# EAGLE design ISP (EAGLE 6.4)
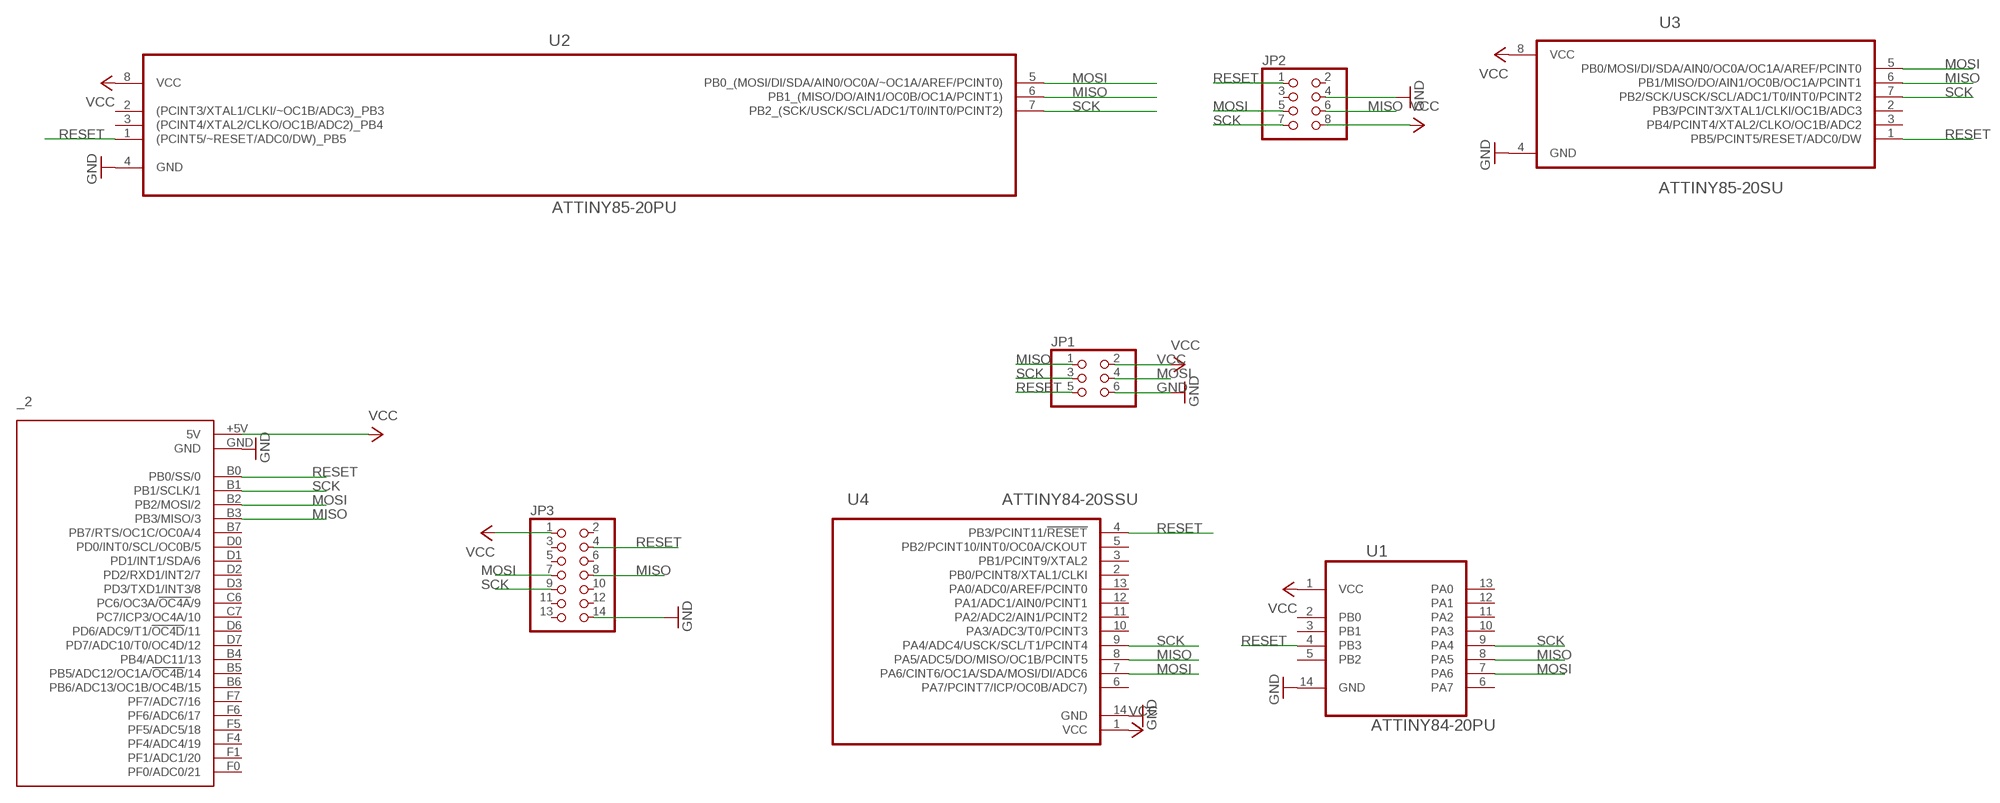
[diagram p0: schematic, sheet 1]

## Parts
_2  TEENSY-OUTER  [TEENSY-OUTER]
JP1  PINHD-2X3  [2X03]
JP2  PINHD-2X4  [2X04]
JP3  PINHD-2X7  [2X07]
U1  ATTINY84-20PU  [DIP254P762X533-14]
U2  ATTINY85-20PU  [DIP254P762X533-8]
U3  ATTINY85-20SU  [SOIC127P798X216-8N]
U4  ATTINY84-20SSU  [SOIC127P600X175-14N]

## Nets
GND: _2.GND JP1.6 JP2.4 JP3.14 U1.14(GND) U2.4(GND) U3.4(GND) U4.14(GND)
MISO: _2.B3(PB3/MISO/3) JP1.1 JP2.6 JP3.8 U1.8(PA5) U2.6(PB1_(MISO/DO/AIN1/OC0B/OC1A/PCINT1)) U3.6(PB1/MISO/DO/AIN1/OC0B/OC1A/PCINT1) U4.8(PA5/ADC5/DO/MISO/OC1B/PCINT5)
MOSI: _2.B2(PB2/MOSI/2) JP1.4 JP2.5 JP3.7 U1.7(PA6) U2.5(PB0_(MOSI/DI/SDA/AIN0/OC0A/~OC1A/AREF/PCINT0)) U3.5(PB0/MOSI/DI/SDA/AIN0/OC0A/OC1A/AREF/PCINT0) U4.7(PA6/CINT6/OC1A/SDA/MOSI/DI/ADC6)
RESET: _2.B0(PB0/SS/0) JP1.5 JP2.1 JP3.4 U1.4(PB3) U2.1((PCINT5/~RESET/ADC0/DW)_PB5) U3.1(PB5/PCINT5/RESET/ADC0/DW) U4.4(PB3/PCINT11/!RESET)
SCK: _2.B1(PB1/SCLK/1) JP1.3 JP2.7 JP3.9 U1.9(PA4) U2.7(PB2_(SCK/USCK/SCL/ADC1/T0/INT0/PCINT2)) U3.7(PB2/SCK/USCK/SCL/ADC1/T0/INT0/PCINT2) U4.9(PA4/ADC4/USCK/SCL/T1/PCINT4)
VCC: _2.+5V(5V) JP1.2 JP2.8 JP3.1 U1.1(VCC) U2.8(VCC) U3.8(VCC) U4.1(VCC)
Unconnected: _2.B4(PB4/ADC11/13) _2.B5(PB5/ADC12/OC1A/!OC4B!/14) _2.B6(PB6/ADC13/OC1B/OC4B/15) _2.B7(PB7/RTS/OC1C/OC0A/4) _2.C6(PC6/OC3A/!OC4A!/9) _2.C7(PC7/ICP3/OC4A/10) _2.D0(PD0/INT0/SCL/OC0B/5) _2.D1(PD1/INT1/SDA/6) _2.D2(PD2/RXD1/INT2/7) _2.D3(PD3/TXD1/INT3/8) _2.D6(PD6/ADC9/T1/!OC4D!/11) _2.D7(PD7/ADC10/T0/OC4D/12) _2.F0(PF0/ADC0/21) _2.F1(PF1/ADC1/20) _2.F4(PF4/ADC4/19) _2.F5(PF5/ADC5/18) _2.F6(PF6/ADC6/17) _2.F7(PF7/ADC7/16) JP2.2 JP2.3 JP3.2 JP3.3 JP3.5 JP3.6 JP3.10 JP3.11 JP3.12 JP3.13 U1.2(PB0) U1.3(PB1) U1.5(PB2) U1.6(PA7) U1.10(PA3) U1.11(PA2) U1.12(PA1) U1.13(PA0) U2.2((PCINT3/XTAL1/CLKI/~OC1B/ADC3)_PB3) U2.3((PCINT4/XTAL2/CLKO/OC1B/ADC2)_PB4) U3.2(PB3/PCINT3/XTAL1/CLKI/OC1B/ADC3) U3.3(PB4/PCINT4/XTAL2/CLKO/OC1B/ADC2) U4.2(PB0/PCINT8/XTAL1/CLKI) U4.3(PB1/PCINT9/XTAL2) U4.5(PB2/PCINT10/INT0/OC0A/CKOUT) U4.6(PA7/PCINT7/ICP/OC0B/ADC7)) U4.10(PA3/ADC3/T0/PCINT3) U4.11(PA2/ADC2/AIN1/PCINT2) U4.12(PA1/ADC1/AIN0/PCINT1) U4.13(PA0/ADC0/AREF/PCINT0)

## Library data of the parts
_2 = MikesParts:TEENSY-OUTER: Teensy 2.0 Original Design by Clint Fisher Modified Design by Tamir Emran Licensed Under Creative Commons Attribution-ShareAlike 3.0 Unported (CC BY-SA 3.0)
JP1 = MikesParts:PINHD-2X3: PIN HEADER
JP2 = MikesParts:PINHD-2X4: PIN HEADER
JP3 = MikesParts:PINHD-2X7: PIN HEADER
U1 = MikesParts:ATTINY84-20PU: 8-bit Microcontroller with In-System Programmable Flash; MPN: ATTINY84-20PU; OC_FARNELL: -; OC_NEWARK: 58M3794; PACKAGE: PDIP-14; SUPPLIER: Atmel
U2 = MikesParts:ATTINY85-20PU: 8-bit Microcontroller with In-System Programmable Flash; MPN: ATTINY85-20PU; OC_FARNELL: 1455162; OC_NEWARK: 58M3796; PACKAGE: PDIP-8; SUPPLIER: Atmel
U3 = MikesParts:ATTINY85-20SU: 8-bit Microcontroller with In-System Programmable Flash; MPN: ATTINY85-20SU; OC_FARNELL: 1455164; OC_NEWARK: 58M3797; PACKAGE: SOIC-8; SUPPLIER: Atmel
U4 = MikesParts:ATTINY84-20SSU: 8-bit Microcontroller with Bytes In-System Programmable Flash; MPN: ATTINY84-20SSU; OC_FARNELL: 1636955; OC_NEWARK: 03P2040; PACKAGE: SOIC-14; SUPPLIER: Atmel

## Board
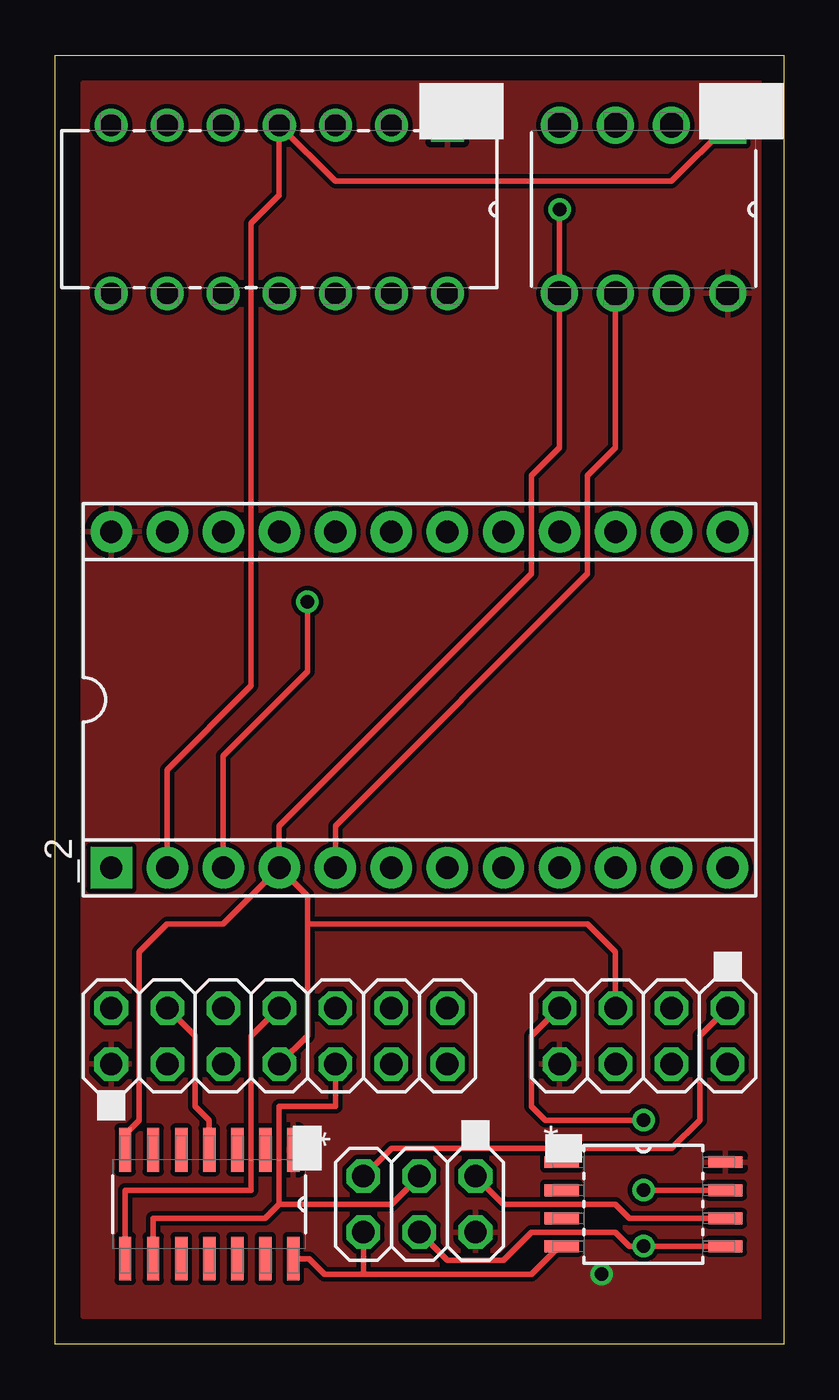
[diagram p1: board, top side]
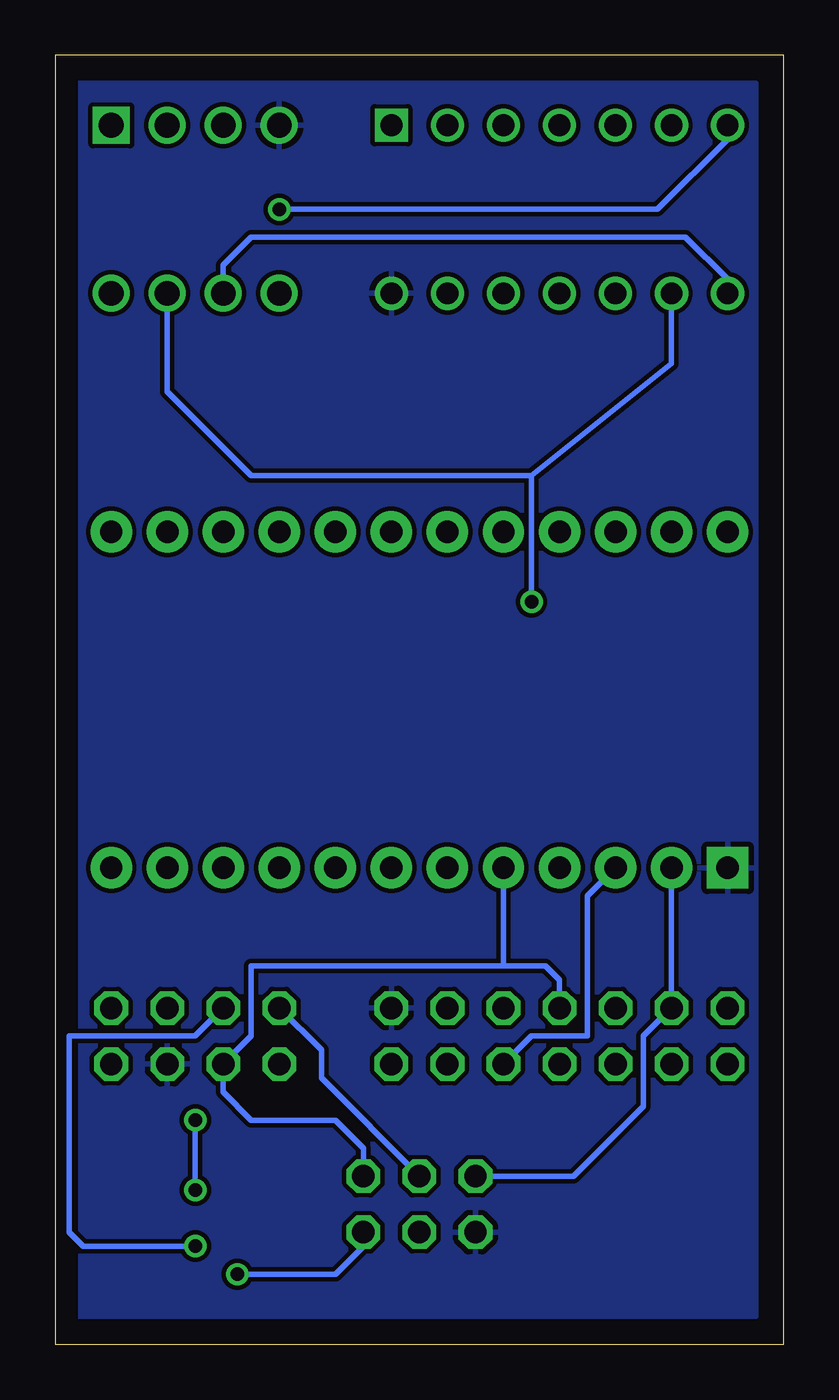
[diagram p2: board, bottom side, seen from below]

Size 33.02 x 58.42 mm. Coordinates in mm from the lower left corner, seen from the top.
Outline: 0,0 0,58.42 33.02,58.42 33.02,0 0,0
Copper layers (1*16): Top 0.035mm / dielectric 1.5mm / Bottom 0.035mm
Design rules "default": minimum track width 10mil, minimum drill 24mil, track to track 8mil, track to pad 8mil, pad to pad 8mil, via to via 8mil, smd to smd 8mil, copper to edge 40mil, drill to drill 8mil, minimum pad ring 10mil, minimum via ring 8mil, stop-mask expansion 4mil, vias tented up to drill 0mil, thermal gap 10mil

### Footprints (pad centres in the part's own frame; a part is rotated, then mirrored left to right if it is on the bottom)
TEENSY-OUTER = drill 1.016 pad 1.88: +5V -13.97,7.62; B0 -11.43,-7.62; B1 -8.89,-7.62; B2 -6.35,-7.62; B3 -3.81,-7.62; B4 8.89,7.62; B5 6.35,7.62; B6 3.81,7.62; B7 -1.27,-7.62; C6 11.43,-7.62; C7 13.97,-7.62; D0 1.27,-7.62; D1 3.81,-7.62; D2 6.35,-7.62; D3 8.89,-7.62; D6 13.97,7.62; D7 11.43,7.62; F0 -11.43,7.62; F1 -8.89,7.62; F4 -6.35,7.62; F5 -3.81,7.62; F6 -1.27,7.62; F7 1.27,7.62 | drill 1.016 pad 1.88 square: GND -13.97,-7.62
2X03 = drill 1.016 octagon: 1 -2.54,-1.27; 2 -2.54,1.27; 3 0,-1.27; 4 0,1.27; 5 2.54,-1.27; 6 2.54,1.27
2X04 = drill 1.016 octagon: 1 -3.81,-1.27; 2 -3.81,1.27; 3 -1.27,-1.27; 4 -1.27,1.27; 5 1.27,-1.27; 6 1.27,1.27; 7 3.81,-1.27; 8 3.81,1.27
2X07 = drill 1.016 octagon: 1 -7.62,-1.27; 2 -7.62,1.27; 3 -5.08,-1.27; 4 -5.08,1.27; 5 -2.54,-1.27; 6 -2.54,1.27; 7 0,-1.27; 8 0,1.27; 9 2.54,-1.27; 10 2.54,1.27; 11 5.08,-1.27; 12 5.08,1.27; 13 7.62,-1.27; 14 7.62,1.27
DIP254P762X533-14 = drill 0.991 square: 1 -7.62,15.24 | drill 0.991: 2 -7.62,12.7; 3 -7.62,10.16; 4 -7.62,7.62; 5 -7.62,5.08; 6 -7.62,2.54; 7 -7.62,0; 8 0,0; 9 0,2.54; 10 0,5.08; 11 0,7.62; 12 0,10.16; 13 0,12.7; 14 0,15.24
DIP254P762X533-8 = drill 1.118 square: 1 -7.62,7.62 | drill 1.118: 2 -7.62,5.08; 3 -7.62,2.54; 4 -7.62,0; 5 0,0; 6 0,2.54; 7 0,5.08; 8 0,7.62
SOIC127P798X216-8N = smd 1.549 x 0.533: 1 -3.708,1.905; 2 -3.708,0.635; 3 -3.708,-0.635; 4 -3.708,-1.905; 5 3.708,-1.905; 6 3.708,-0.635; 7 3.708,0.635; 8 3.708,1.905
SOIC127P600X175-14N = smd 1.981 x 0.559: 1 -2.464,3.81; 2 -2.464,2.54; 3 -2.464,1.27; 4 -2.464,0; 5 -2.464,-1.27; 6 -2.464,-2.54; 7 -2.464,-3.81; 8 2.464,-3.81; 9 2.464,-2.54; 10 2.464,-1.27; 11 2.464,0; 12 2.464,1.27; 13 2.464,2.54; 14 2.464,3.81

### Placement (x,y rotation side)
_2  16.51,29.21 0 top
JP1  16.51,6.35 180 top
JP2  26.67,13.97 180 top
JP3  10.16,13.97 0 top
U1  2.54,47.62 270 top
U2  22.86,47.62 270 top
U3  26.67,6.35 0 top
U4  6.98,6.35 270 top

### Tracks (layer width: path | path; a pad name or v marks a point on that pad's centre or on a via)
GND
  Top 0.254: U3.4 22.86,4.45 21.59,3.17 13.97,3.17 | 13.97,3.17 12.22,3.17 11.51,3.89 U4.14 | JP1.6 13.97,3.17
  pour Bottom: 1.27,57.15 33.02,57.15 33.02,1.27 1.27,1.27
MISO
  Top 0.254: U4.8 3.17,6.98 8.89,6.98 8.89,13.97 JP3.8 | U3.6 26.04,5.71 25.4,6.35 20.32,6.35 JP1.1 | _2.B3 12.7,23.5 24.13,34.93 24.13,39.37 25.4,40.64 U2.6
  Bottom 0.254: _2.B3 12.7,17.14 | JP1.1 19.05,8.89 20.32,10.16 24.13,10.16 25.4,11.43 JP2.6 24.13,13.97 24.13,17.14 12.7,17.14 | U1.8 2.54,48.26 4.45,50.17 24.13,50.17 25.4,48.9 U2.6 | JP3.8 10.16,16.51 10.79,17.14 12.7,17.14
MOSI  (via drill 0.61)
  Top 0.254: U4.7 3.17,9.53 3.81,10.16 3.81,17.78 5.08,19.05 7.62,19.05 _2.B2 | JP1.4 17.78,3.81 20.32,3.81 21.59,5.08 25.4,5.08 26.04,4.45 v26.67,4.45 U3.5 30.48,4.34 | JP3.7 11.43,13.97 11.43,19.05 | 11.43,19.05 11.43,20.32 _2.B2 | 11.43,19.05 24.13,19.05 25.4,17.78 JP2.5 | v22.86,51.44 U2.5 22.86,40.64 21.59,39.37 21.59,34.93 10.16,23.5 _2.B2
  Bottom 0.254: JP2.5 26.67,13.97 32.38,13.97 32.38,5.08 31.75,4.45 v26.67,4.45 | U1.7 2.54,54.61 5.71,51.44 v22.86,51.44
RESET
  Top 0.254: JP3.4 6.35,13.97 6.35,10.79 6.98,10.16 U4.4 | JP1.5 15.24,8.89 22.86,8.89 | 22.86,8.89 27.94,8.89 29.21,10.16 29.21,13.97 JP2.1 | U3.1 22.96,8.79 22.86,8.89 | U2.1 27.94,52.71 12.7,52.71 U1.4 10.16,52.07 8.89,50.8 8.89,29.84 5.08,26.04 _2.B0
  Bottom 0.254: _2.B0 JP3.4 6.35,13.97 6.35,10.79 9.53,7.62 JP1.5
SCK  (via drill 0.61)
  Top 0.254: U4.9 4.45,5.71 9.53,5.71 10.16,6.35 | 10.16,6.35 10.16,10.79 12.7,10.79 JP3.9 | U3.7 v26.67,6.98 | JP1.3 15.24,6.35 10.16,6.35 | JP2.7 21.59,13.97 21.59,10.79 22.22,10.16 v26.67,10.16 | _2.B1 7.62,26.67 11.43,30.48 v11.43,33.66
  Bottom 0.254: JP3.9 11.43,13.97 8.89,13.97 8.89,20.32 _2.B1 | v26.67,6.98 v26.67,10.16 | JP2.7 20.95,13.33 20.95,12.06 JP1.3 | U1.9 5.08,44.45 11.43,39.37 | 11.43,39.37 v11.43,33.66 | U2.7 27.94,43.18 24.13,39.37 11.43,39.37
VCC  (via drill 0.61)
  Bottom 0.254: JP1.2 19.05,4.45 20.32,3.17 v24.77,3.17
  pour Top: 1.27,1.27 1.27,57.15 33.02,57.15 33.02,1.27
